[IBIS Ver]   3.2
[Comment Char]   |_char
[File Name]   sprm286.ibs
[File Rev]   1.0
[Date]   November 15, 2006
[Source]   From Ansoft Q3D ver 7.0 result.
[Notes]
[Disclaimer]
[Copyright]
[Component]   F2802PZ
[Manufacturer]   ti
[Package]
| variable   typ   min   max
R_pkg   2.30437e-001  2.08189e-001  2.60722e-001
L_pkg   4.72707e-009  4.16780e-009  5.57252e-009
C_pkg   7.13737e-013  6.35506e-013  8.14892e-013
[Pin]  signal_name   model_name   R_pin   L_pin   C_pin
01   GP_IO[12]  BC3350AFHYPU_3P3PU   2.41885E-01  5.15245E-09  7.14883E-13
02   VSS   NC   2.34357E-01  4.94630E-09  7.96557E-13
03   VDDIO   NC   2.46145E-01  5.01747E-09  7.72000E-13
04   GP_IO[29]  BC3325CFHYPU_3P3PU   2.60722E-01  5.07403E-09  7.81142E-13
05   GP_IO[33]  BC3350AFHYPU_3P3PU   2.52780E-01  4.93394E-09  7.70698E-13
06   GP_IO[30]  BC3325CFHYPU_3P3PU   2.43329E-01  4.79386E-09  7.44586E-13
07   GP_IO[31]  BC3325CFHYPU_3P3PU   2.35995E-01  4.68483E-09  7.19311E-13
08   GP_IO[14]  BC3350AFHYPU_3P3PU   2.29764E-01  4.57742E-09  6.99571E-13
09   GP_IO[15]  BC3350AFHYPU_3P3PU   2.24030E-01  4.50311E-09  6.77180E-13
10   VDD   NC   2.19563E-01  4.45501E-09  6.43759E-13
11   VSS   NC   2.47586E-01  4.68056E-09  6.54842E-13
12   VDD1   NC   2.41580E-01  4.62250E-09  6.57690E-13
13   VSS1   NC   2.35066E-01  4.55577E-09  6.56277E-13
14   VSSA2   NC   2.29936E-01  4.53126E-09  6.48777E-13
15   VDDAFL2   NC   2.23371E-01  4.50511E-09  6.47774E-13
16   ADCINA[7]   NC   2.21960E-01  4.53610E-09  6.57212E-13
17   ADCINA[6]   NC   2.18585E-01  4.55776E-09  6.75450E-13
18   ADCINA[5]   NC   2.15805E-01  4.59790E-09  6.88161E-13
19   ADCINA[4]   NC   2.15842E-01  4.67531E-09  7.03692E-13
20   ADCINA[3]   NC   2.15931E-01  4.75864E-09  7.23998E-13
21   ADCINA[2]   NC   2.18706E-01  4.87599E-09  7.42438E-13
22   ADCINA[1]   NC   2.22439E-01  5.01168E-09  7.61304E-13
23   ADCINA[0]   NC   2.28012E-01  5.16249E-09  7.86322E-13
24   ADCLO   NC   2.36367E-01  5.33365E-09  8.10938E-13
25   VSSA11   NC   2.42705E-01  5.57252E-09  7.25356E-13
26   VDDAFL11   NC   2.41927E-01  5.39649E-09  7.33227E-13
27   ADCINB[0]   NC   2.31818E-01  5.08323E-09  8.14446E-13
28   ADCINB[1]   NC   2.23112E-01  4.87963E-09  7.83445E-13
29   ADCINB[2]   NC   2.16528E-01  4.66967E-09  7.60019E-13
30   ADCINB[3]   NC   2.11164E-01  4.51040E-09  7.35949E-13
31   ADCINB[4]   NC   2.08744E-01  4.38092E-09  7.14391E-13
32   ADCINB[5]   NC   2.08189E-01  4.29268E-09  6.97473E-13
33   ADCINB[6]   NC   2.09857E-01  4.22696E-09  6.83167E-13
34   ADCINB[7]   NC   2.11840E-01  4.18683E-09  6.69921E-13
35   ADCREFIN   NC   2.14738E-01  4.16780E-09  6.59648E-13
36   ADCREFM   NC   2.20908E-01  4.17569E-09  6.51875E-13
37   ADCREFP   NC   2.25652E-01  4.21926E-09  6.35506E-13
38   ADCRESEXT   NC   2.23711E-01  4.19946E-09  6.36197E-13
39   VSSA1   NC   2.30139E-01  4.28338E-09  6.48736E-13
40   VDDA1   NC   2.37075E-01  4.38588E-09  6.66868E-13
41   VSS   NC   2.43391E-01  4.53286E-09  6.69682E-13
42   VDD   NC   2.29248E-01  4.46007E-09  6.72298E-13
43   GP_IO[34]  BC3350AFHYPU_3P3PU   2.36981E-01  4.61397E-09  6.92865E-13
44   GP_IO[1]   BC3350AFHYPU_3P3PU   2.29704E-01  4.61554E-09  7.08075E-13
45   GP_IO[2]   BC3350AFHYPU_3P3PU   2.39434E-01  4.79910E-09  7.47205E-13
46   VDDIO   NC   2.48025E-01  5.02376E-09  7.57526E-13
47   GP_IO[0]   BC3350AFHYPU_3P3PU   2.34680E-01  4.97791E-09  7.66837E-13
48   GP_IO[3]   BC3350AFHYPU_3P3PU   2.46329E-01  5.22361E-09  8.04871E-13
49   VSS   NC   2.56466E-01  5.47475E-09  8.14892E-13
50   GP_IO[16] BC3350AFHYPU_3P3PU   2.39732E-01  5.45793E-09  7.01816E-13
51   GP_IO[4]  BC3350AFHYPU_3P3PU   2.43299E-01  5.12464E-09  7.17205E-13
52   GP_IO[17] BC3350AFHYPU_3P3PU   2.34663E-01  4.90755E-09  8.10107E-13
53   GP_IO[5]  BC3350AFHYPU_3P3PU   2.27934E-01  4.79084E-09  7.88169E-13
54   GP_IO[18] BC3350AFHYPU_3P3PU   2.21487E-01  4.66973E-09  7.63683E-13
55   VSS   NC   2.16388E-01  4.59009E-09  7.29478E-13
56   GP_IO[6]  BC3350AFHYPU_3P3PU   2.20058E-01  4.57300E-09  7.12932E-13
57   GP_IO[19] BC3350AFHYPU_3P3PU   2.18566E-01  4.49925E-09  7.09697E-13
58   GP_IO[7]  BC3350AFHYPU_3P3PU   2.16607E-01  4.44809E-09  6.90626E-13
59   VDD   NC   2.15254E-01  4.43939E-09  6.58148E-13
60   GP_IO[8]  BC3350AFHYPU_3P3PU   2.15334E-01  4.40433E-09  6.41439E-13
61   GP_IO[9]  BC3350AFHYPU_3P3PU   2.16208E-01  4.39821E-09  6.43114E-13
62   VSS   NC   2.17947E-01  4.42195E-09  6.25612E-13
63   GP_IO[20] BC3350AFHYPU_3P3PU   2.16379E-01  4.39288E-09  6.25676E-13
64   GP_IO[10] BC3350AFHYPU_3P3PU   2.17555E-01  4.44649E-09  6.33537E-13
65   VDDIO   NC   2.18499E-01  4.49762E-09  6.31103E-13
66   XCLKOUT   BC3325CF_3P3PU   2.15554E-01  4.50560E-09  6.37936E-13
67   GP_IO[21] BC3350AFHYPU_3P3PU   2.18252E-01  4.57466E-09  6.68273E-13
68   VDD   NC   2.20793E-01  4.67924E-09  6.79227E-13
69   VSS   NC   2.16026E-01  4.69108E-09  6.77337E-13
70   GP_IO[11] BC3350AFHYPU_3P3PU   2.16647E-01  4.71155E-09  7.13725E-13
71   GP_IO[22] BC3350AFHYPU_3P3PU   2.18668E-01  4.81184E-09  7.42610E-13
72   GP_IO[23] BC3350AFHYPU_3P3PU   2.21167E-01  4.93087E-09  7.61343E-13
73   TDI   IC33FFSHYPU_3P3PU   2.27003E-01  5.09516E-09  7.84184E-13
74   TMS   IC33FFSHYPU_3P3PU   2.35833E-01  5.26915E-09  8.12419E-13
75   TCK   IC33FFSHYPU_3P3PU   2.44266E-01  5.53529E-09  7.26831E-13
76   TDO   OC3325CF_3P3   2.41553E-01  5.34261E-09  7.19286E-13
77   VSS   NC   2.32208E-01  5.05829E-09  7.97518E-13
78   XRSn   BC3350BFODHYPU_3P3PU   2.35799E-01  5.01747E-09  7.82884E-13
79   GP_IO[27] BC3350AFHYPU_3P3PU   2.28095E-01  4.79742E-09  7.71509E-13
80   EMU0   BC3325CFHYPU_3P3PU   2.19735E-01  4.59334E-09  7.43946E-13
81   EMU1   BC3325CFHYPU_3P3PU   2.13581E-01  4.44129E-09  7.16783E-13
82   VDDIO   NC   2.09468E-01  4.31678E-09  6.88411E-13
83   GP_IO[24] BC3350AFHYPU_3P3PU   2.13253E-01  4.29676E-09  6.77699E-13
84   TRSTn   IC33FFSHYPD_3P3PD   2.10840E-01  4.19129E-09  6.72068E-13
85   VDD   NC   2.08312E-01  4.11081E-09  6.43567E-13
86   X2   NC   2.08945E-01  4.08812E-09  6.31887E-13
87   VSS   NC   2.09662E-01  4.06013E-09  6.35551E-13
88   X1   NC   2.10747E-01  4.04716E-09  6.39624E-13
89   VSS   NC   2.14839E-01  4.10696E-09  6.40567E-13
90   XCLKIN   IC33FFSHY_3P3   2.17217E-01  4.17857E-09  6.38439E-13
91   GP_IO[25] BC3350AFHYPU_3P3PU   2.12121E-01  4.19716E-09  6.29643E-13
92   GP_IO[28] BC3325CFHYPU_3P3PU   2.10521E-01  4.22870E-09  6.45810E-13
93   VDD   NC   2.09838E-01  4.29298E-09  6.61723E-13
94   VSS   NC   2.08411E-01  4.34767E-09  6.83282E-13
95   GP_IO[13] BC3350AFHYPU_3P3PU   2.11594E-01  4.46074E-09  7.09048E-13
96   VDD3V   NC   2.14577E-01  4.59443E-09  7.38105E-13
97   TEST1   NC   2.21880E-01  4.78210E-09  7.69895E-13
98   TEST2   NC   2.30305E-01  5.01868E-09  7.81859E-13
99   GP_IO[26] BC3350AFHYPU_3P3PU   2.30319E-01  5.12357E-09  8.00732E-13
100   GP_IO[32] BC3350AFHYPU_3P3PU   2.40060E-01  5.43681E-09  7.18705E-13
[Define Package Model]  pz_shakti
[Manufacturer]   ti
[OEM]   xyz
[Description]  None
[Number Of Pins]  100
[Pin Numbers]
01   | 01 = P001
02   | 02 = P002
03   | 03 = P003
04   | 04 = P004
05   | 05 = P005
06   | 06 = P006
07   | 07 = P007
08   | 08 = P008
09   | 09 = P009
10   | 10 = P010
11   | 11 = P011
12   | 12 = P012
13   | 13 = P013
14   | 14 = P014
15   | 15 = P015
16   | 16 = P016
17   | 17 = P017
18   | 18 = P018
19   | 19 = P019
20   | 20 = P020
21   | 21 = P021
22   | 22 = P022
23   | 23 = P023
24   | 24 = P024
25   | 25 = P025
26   | 26 = P026
27   | 27 = P027
28   | 28 = P028
29   | 29 = P029
30   | 30 = P030
31   | 31 = P031
32   | 32 = P032
33   | 33 = P033
34   | 34 = P034
35   | 35 = P035
36   | 36 = P036
37   | 37 = P037
38   | 38 = P038
39   | 39 = P039
40   | 40 = P040
41   | 41 = P041
42   | 42 = P042
43   | 43 = P043
44   | 44 = P044
45   | 45 = P045
46   | 46 = P046
47   | 47 = P047
48   | 48 = P048
49   | 49 = P049
50   | 50 = P050
51   | 51 = P051
52   | 52 = P052
53   | 53 = P053
54   | 54 = P054
55   | 55 = P055
56   | 56 = P056
57   | 57 = P057
58   | 58 = P058
59   | 59 = P059
60   | 60 = P060
61   | 61 = P061
62   | 62 = P062
63   | 63 = P063
64   | 64 = P064
65   | 65 = P065
66   | 66 = P066
67   | 67 = P067
68   | 68 = P068
69   | 69 = P069
70   | 70 = P070
71   | 71 = P071
72   | 72 = P072
73   | 73 = P073
74   | 74 = P074
75   | 75 = P075
76   | 76 = P076
77   | 77 = P077
78   | 78 = P078
79   | 79 = P079
80   | 80 = P080
81   | 81 = P081
82   | 82 = P082
83   | 83 = P083
84   | 84 = P084
85   | 85 = P085
86   | 86 = P086
87   | 87 = P087
88   | 88 = P088
89   | 89 = P089
90   | 90 = P090
91   | 91 = P091
92   | 92 = P092
93   | 93 = P093
94   | 94 = P094
95   | 95 = P095
96   | 96 = P096
97   | 97 = P097
98   | 98 = P098
99   | 99 = P099
100   | 100 = P100
[Model Data]
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[End Model Data]
[End Package Model]
|   Component BC3350AFHYPU
[Component]   BC3350AFHYPU
[Manufacturer]   Texas Instruments.
[Package]
| variable   typ   min   max
R_pkg   0.000   0.000   0.000
L_pkg   0.000H   0.000H   0.000H
C_pkg   0.000F   0.000F   0.000F
[Pin]  signal_name   model_name   R_pin   L_pin   C_pin
PAD   PAD   BC3350AFHYPU_3P3PU
| A   A   dummy
| GZ   GZ   dummy
| Y   Y   dummy
VSSS   VSSS   GND
VDDS   VDDS   POWER
[Model Selector]  BC3350AFHYPU
BC3350AFHYPU_2P5PU   cell   VDDS=2.5V(typ)  PI=0
BC3350AFHYPU_2P5PUZ  cell   VDDS=2.5V(typ)  PI=1
BC3350AFHYPU_3P3PU   cell   VDDS=3.3V(typ)  PI=0
BC3350AFHYPU_3P3PUZ  cell   VDDS=3.3V(typ)  PI=1
|   Component BC3325CFHYPU
[Component]   BC3325CFHYPU
[Manufacturer]   Texas Instruments.
[Package]
| variable   typ   min   max
R_pkg   0.000   0.000   0.000
L_pkg   0.000H   0.000H   0.000H
C_pkg   0.000F   0.000F   0.000F
[Pin]  signal_name   model_name   R_pin   L_pin   C_pin
PAD   PAD   BC3325CFHYPU_3P3PU
| A   A   dummy
| GZ   GZ   dummy
| Y   Y   dummy
VSSS   VSSS   GND
VDDS   VDDS   POWER
[Model Selector]   BC3325CFHYPU
BC3325CFHYPU_2P5PU   cell  VDDS=2.75(TYP)  PI=0
BC3325CFHYPU_2P5PUZ   cell  VDDS=2.75(TYP)  PI=1
BC3325CFHYPU_3P3PU   cell  VDDS=3.3(TYP)  PI=0
BC3325CFHYPU_3P3PUZ   cell  VDDS=3.3(TYP)  PI=1
|   Component OC3325CF
[Component]   OC3325CF
[Manufacturer]   Texas Instruments.
[Package]
| variable   typ   min   max
R_pkg   0.000   0.000   0.000
L_pkg   0.000H   0.000H   0.000H
C_pkg   0.000F   0.000F   0.000F
[Pin]  signal_name   model_name   R_pin   L_pin   C_pin
PAD   PAD   OC3325CF_3P3
| A   A   dummy
| GZ   GZ   dummy
VDDS   VDDS   POWER
VSSS   VSSS   GND
VSS   VSS   GND
[Model Selector]   OC3325CF
OC3325CF_2P5  cell VDDS=2.5V(typ)
OC3325CF_2P7  cell VDDS=2.75V(typ)
OC3325CF_3P3  cell VDDS=3.3V(typ)
|   Component BC3350BFODHYPU
[Component]   BC3350BFODHYPU
[Manufacturer]   Texas Instruments.
[Package]
| variable   typ   min   max
R_pkg   0.000   0.000   0.000
L_pkg   0.000H   0.000H   0.000H
C_pkg   0.000F   0.000F   0.000F
[Pin]  signal_name   model_name   R_pin   L_pin   C_pin
PAD   PAD   BC3350BFODHYPU_3P3PU
| A   A   dummy
| GZ   GZ   dummy
| Y   Y   dummy
VSSS   VSSS   GND
VDDS   VDDS   POWER
[Model Selector]   BC3350BFODHYPU
BC3350BFODHYPU_2P5PU   cell   VDDS=2.75(TYP)
BC3350BFODHYPU_2P5PZ   cell   VDDS=2.75(TYP)
BC3350BFODHYPU_3P3PU   cell   VDDS=3.3(TYP)
BC3350BFODHYPU_3P3PZ   cell   VDDS=3.3(TYP)
|   Component IC33FFSHYPD
[Component]   IC33FFSHYPD
[Manufacturer]   Texas Instruments.
[Package]
| variable   typ   min   max
R_pkg   0.000   0.000   0.000
L_pkg   0.000H   0.000H   0.000H
C_pkg   0.000F   0.000F   0.000F
[Pin]  signal_name   model_name   R_pin   L_pin   C_pin
PAD   PAD   IC33FFSHYPD_3P3PD
| Y   Y   dummy
VSS   VSS   GND
VDDS   VDDS   POWER
[Model Selector]  IC33FFSHYPD
IC33FFSHYPD_2P7PD   cell with PI=0 and VDDS as 2.75(typ)
IC33FFSHYPD_2P7PDZ   cell with PI=1 and VDDS as 2.75(typ)
IC33FFSHYPD_3P3PD   cell with PI=0 and VDDS as 3.3(typ)
IC33FFSHYPD_3P3PDZ   cell with PI=1 and VDDS as 3.3(typ)
|   Component BC3325CF
[Component]   BC3325CF
[Manufacturer]   Texas Instruments.
[Package]
| variable   typ   min   max
R_pkg   0.000   0.000   0.000
L_pkg   0.000H   0.000H   0.000H
C_pkg   0.000F   0.000F   0.000F
[Pin]  signal_name   model_name   R_pin   L_pin   C_pin
PAD   PAD   BC3325CF_3P3PU
| A   A   dummy
| GZ   GZ   dummy
| Y   Y   dummy
VSSS   VSSS   GND
VDDS   VDDS   POWER
[Model Selector]  BC3325CF
BC3325CF_2P5PU  cell   VDDS=2.75V(typ)
BC3325CF_3P3PU  cell   VDDS=3.30V(typ)
|   Component IC33FFSHYPU
[Component]   IC33FFSHYPU
[Manufacturer]   Texas Instruments.
[Package]
| variable   typ   min   max
R_pkg   0.000   0.000   0.000
L_pkg   0.000H   0.000H   0.000H
C_pkg   0.000F   0.000F   0.000F
[Pin]  signal_name   model_name   R_pin   L_pin   C_pin
PAD   PAD   IC33FFSHYPU_3P3PU
| Y   Y   dummy
VSS   VSS   GND
VDDS   VDDS   POWER
[Model Selector]  IC33FFSHYPU
IC33FFSHYPU_2P5PU   cell with PI=0 VDDS=2.5(typ)
IC33FFSHYPU_2P5PUZ   cell with PI=1 VDDS=2.5(typ)
IC33FFSHYPU_2P7PU   cell with PI=0 VDDS=2.7(typ)
IC33FFSHYPU_2P7PUZ   cell with PI=1 VDDS=2.7(typ)
IC33FFSHYPU_3P3PU   cell with PI=0 VDDS=3.3(typ)
IC33FFSHYPU_3P3PUZ   cell with PI=1 VDDS=3.3(typ)
|   Component IC33FFSHY
[Component]   IC33FFSHY
[Manufacturer]   Texas Instruments.
[Package]
| variable   typ   min   max
R_pkg   0.000   0.000   0.000
L_pkg   0.000H   0.000H   0.000H
C_pkg   0.000F   0.000F   0.000F
[Pin]  signal_name   model_name   R_pin   L_pin   C_pin
PAD   PAD   IC33FFSHY_3P3
| Y   Y   dummy
VSS   VSS   GND
VDDS   VDDS   POWER
[Model Selector]  IC33FFSHY
IC33FFSHY_2P5   cell with VDDS=2.5(NOM)
IC33FFSHY_2P7   cell with VDDS=2.7(NOM)
IC33FFSHY_3P3   cell with VDDS=3.3(NOM)
| Models and submodels in the file (30): BC3350AFHYPU_2P5PU (I/O), BC3350AFHYPU_2P5PUZ (I/O), BC3350AFHYPU_3P3PU (I/O), BC3350AFHYPU_3P3PUZ (I/O), BC3325CFHYPU_2P5PU (I/O), BC3325CFHYPU_2P5PUZ (I/O), BC3325CFHYPU_3P3PU (I/O), BC3325CFHYPU_3P3PUZ (I/O), OC3325CF_2P5 (3-state), OC3325CF_2P7 (3-state), OC3325CF_3P3 (3-state), BC3350BFODHYPU_2P5PU (I/O_open_drain), BC3350BFODHYPU_2P5PZ (I/O_open_drain), BC3350BFODHYPU_3P3PU (I/O_open_drain), BC3350BFODHYPU_3P3PZ (I/O_open_drain), IC33FFSHYPD_2P7PD (Input), IC33FFSHYPD_2P7PDZ (Input), IC33FFSHYPD_3P3PD (Input), IC33FFSHYPD_3P3PDZ (Input), BC3325CF_2P5PU (I/O), BC3325CF_3P3PU (I/O), IC33FFSHYPU_2P5PU (Input), IC33FFSHYPU_2P5PUZ (Input), IC33FFSHYPU_2P7PU (Input), IC33FFSHYPU_2P7PUZ (Input), IC33FFSHYPU_3P3PU (Input), IC33FFSHYPU_3P3PUZ (Input), IC33FFSHY_2P5 (Input), IC33FFSHY_2P7 (Input), IC33FFSHY_3P3 (Input)
